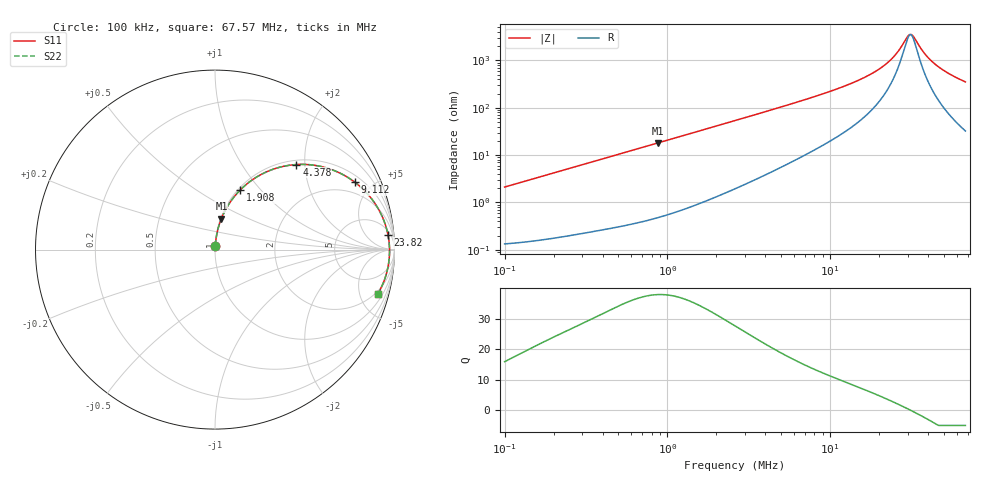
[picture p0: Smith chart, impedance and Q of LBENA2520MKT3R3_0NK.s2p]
! LBENA2520MKT3R3_0NK  S-PARAMETER MODEL  ( General Type )
! Model Generated by TAIYO YUDEN Corporation (http://www.ty-top.com)
! Version 1.0
! TAIYO YUDEN Control No. 220120
! Copyright(c) 2022 TAIYO YUDEN CO.,LTD. All Rights Reserved.
! Product Description (link to TY-COMPAS)
! https://ds.yuden.co.jp/TYCOMPAS/or/detail?pn=LBENA2520MKT3R3M0NK&u=M
! Products Name : Inductors
! Characteristics :
!  Inductance : 3.3 uH , SRF(min) : -Hz , DC Resistance(max) : 0.131 Ohm
!  Rated Current : Saturation :2300 mA , Temp Rise : 1800 mA
!  Case Size : 2.5 x 2.0 / 0.098 x 0.079 [mm/inch] , Thickness : 1.2 / 0.047 [mm/inch]
!  (Conditions: Temperature = 25 degC , DC Bias Current/Voltage = 0A / 0V)
! External Node Assignments :
!  1  o---GGG---o  2
! GND o---------o GND
! Frequency Range : 0.1MHz  -  67.570357MHz  [ 402 STEP ]
# MHz S RI R 50
! Freq[MHz].  S11 Real  S11 Imag  S21 Real  S21 Imag  S12 Real  S12 Imag  S22 Real  S22 Imag
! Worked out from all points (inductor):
!   401 points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, 100 kHz to 67.57 MHz, reference 50 ohm
!   read as one part in series: L = 3.36 uH near 103.3 kHz
!   highest Q = 37.8 at 872.8 kHz (marker M1), where L = 3.29 uH
!   self-resonance near 31.07 MHz
!   S11 on the Smith chart (normalised r, x): 100 kHz: 1.00, +0.04; 1.908 MHz: 1.02, +0.79; 4.378 MHz: 1.09, +1.81; 9.112 MHz: 1.33, +3.97; 23.82 MHz: 8, +20; 67.57 MHz: 1.65, -7.01
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0.1  0.00177 0.0211  0.9982 -0.0211  0.9982 -0.0211  0.00177 0.0211
0.297841  0.00603 0.0618  0.994 -0.0618  0.994 -0.0618  0.00603 0.0618
0.872758  0.0359 0.1732  0.9641 -0.1732  0.9641 -0.1732  0.0359 0.1732
0.887091  0.0369 0.1758  0.9631 -0.1758  0.9631 -0.1758  0.0369 0.1758
1.907501  0.1416 0.3333  0.8584 -0.3333  0.8584 -0.3333  0.1416 0.3333
2.59943  0.2311 0.4038  0.7689 -0.4038  0.7689 -0.4038  0.2311 0.4038
4.377827  0.4539 0.474  0.5461 -0.474  0.5461 -0.474  0.4539 0.474
7.742162  0.7191 0.4144  0.2809 -0.4144  0.2809 -0.4144  0.7191 0.4144
9.111842  0.7804 0.3746  0.2196 -0.3746  0.2196 -0.3746  0.7804 0.3746
12.41708  0.8709 0.2852  0.1291 -0.2852  0.1291 -0.2852  0.8709 0.2852
16.11424  0.9221 0.2043  0.0779 -0.2043  0.0779 -0.2043  0.9221 0.2043
19.59307  0.9477 0.1431  0.0523 -0.1431  0.0523 -0.1431  0.9477 0.1431
23.05932  0.9618 0.0924  0.0382 -0.0924  0.0382 -0.0924  0.9618 0.0924
23.82293  0.9639 0.0823  0.0361 -0.0823  0.0361 -0.0823  0.9639 0.0823
26.26888  0.9688 0.052  0.0312 -0.052  0.0312 -0.052  0.9688 0.052
29.92517  0.9722 0.0116  0.0278 -0.0116  0.0278 -0.0116  0.9722 0.0116
31.42388  0.9726 -0.00356  0.0274 0.00356  0.0274 0.00356  0.9726 -0.00356
32.99765  0.9724 -0.0188  0.0276 0.0188  0.0276 0.0188  0.9724 -0.0188
38.20784  0.9691 -0.0647  0.0309 0.0647  0.0309 0.0647  0.9691 -0.0647
43.52589  0.9621 -0.106  0.0379 0.106  0.0379 0.106  0.9621 -0.106
52.9225  0.9439 -0.1692  0.0561 0.1692  0.0561 0.1692  0.9439 -0.1692
67.57036  0.9058 -0.2497  0.0942 0.2497  0.0942 0.2497  0.9058 -0.2497
